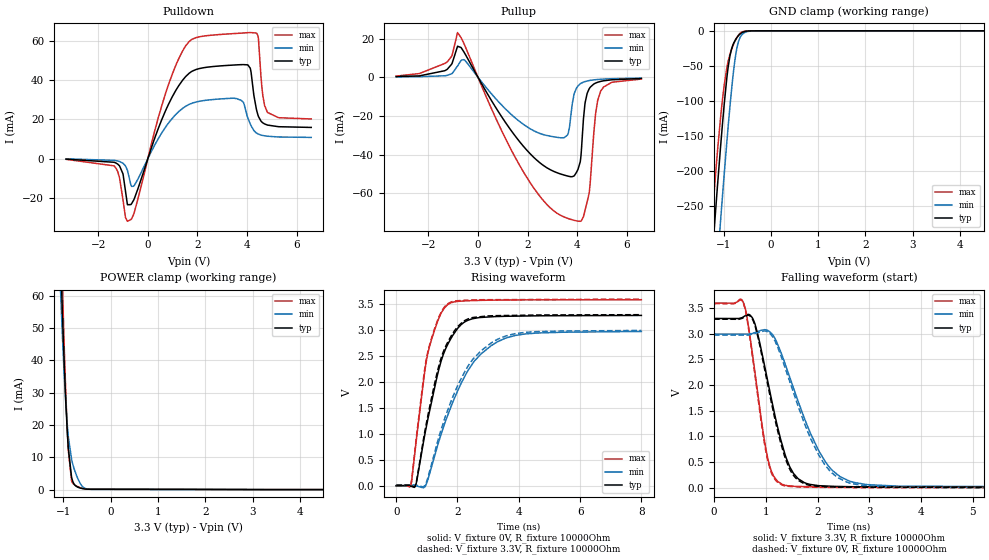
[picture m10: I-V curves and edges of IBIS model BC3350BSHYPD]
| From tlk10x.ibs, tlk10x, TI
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|   Model
[Model]   BC3350BSHYPD
Model_type   I/O
Polarity   Non-Inverting
Enable   Active-Low
Vinl = 0.99
Vinh = 2.31
Vmeas = 1.65
Vref = 1.65
Cref = 1pF
Rref = 10000
|   typ   min   max
C_comp   1.945pF   1.862pF   2.001pF
[Voltage Range]   3.3   3   3.6
[Temperature Range]   25   125   -40
[Pullup Reference]   3.3   3   3.6
[Pulldown Reference]   -0   -0   -0
[Power Clamp Reference]   3.3   3   3.6
[GND Clamp Reference]   -0   -0   -0
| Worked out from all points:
|   slope of the pulldown table from 0 to 0.495 V, typ, clamps not added: 27.8 ohm
|   slope of the pullup table from 0 to 0.495 V, typ, clamps not added: 45 ohm
|   GND clamp passes 1 mA (typ) near -0.55 V on its own axis
|   POWER clamp passes 1 mA (typ) near -0.72 V on its own axis
|   falling waveform, V_fixture 3.3V, R_fixture 10000Ohm: 20-80 % time 445ps typ, 712ps min, 304ps max; typ from 3.29 V to 0.009 V
|   rising waveform, V_fixture 0V, R_fixture 10000Ohm: 20-80 % time 768ps typ, 1.26ns min, 555ps max; typ from 0 V to 3.28 V
|   rising waveform, V_fixture 3.3V, R_fixture 10000Ohm: 20-80 % time 752ps typ, 1.21ns min, 552ps max; typ from 0.009 V to 3.29 V
|   falling waveform, V_fixture 0V, R_fixture 10000Ohm: 20-80 % time 438ps typ, 692ps min, 301ps max; typ from 3.28 V to 0 V
[Pulldown]
|   Voltage   I(typ)   I(min)   I(max)
-3.3V     -306.9uA   -177.2uA   -405.8uA
-1.36V    -1.92mA    -935.1uA   -3.757mA
-904.2mV  -16.59mA   -3.769mA   -30.07mA
-676.5mV  -23.41mA   -13.77mA   -31.09mA
976.8mV   31.4mA     20.44mA    42.88mA
2.224V    46.37mA    29.58mA    62.55mA
3.749V    47.99mA    29.83mA    64.09mA
4.036V    47.8mA     20.63mA    64.34mA
4.392V    24.41mA    12.94mA    64.04mA
4.64V     18.21mA    11.76mA    31.98mA
4.818V    17.14mA    11.41mA    23.72mA
6.59V     15.9mA     10.79mA    20.22mA
[GND Clamp]
|   Voltage   I(typ)   I(min)   I(max)
-3.3V     -2.327A    -2.431A    -2.267A
-1.251V   -331.9mA   -441.7mA   -275.1mA
-1.142V   -233.8mA   -342.1mA   -183mA
-1.063V   -165.7mA   -271.4mA   -124mA
-993.3mV  -110.6mA   -211.3mA   -81.83mA
-933.9mV  -69.64mA   -161.9mA   -54.33mA
-864.6mV  -35.7mA    -108.2mA   -33.42mA
-795.3mV  -19.15mA   -61.62mA   -20.36mA
-735.9mV  -11.53mA   -31.57mA   -11.73mA
-676.5mV  -6.269mA   -13.91mA   -5.467mA
-597.3mV  -2.127mA   -4.66mA    -1.311mA
6.59V     0A         0A         0A
[Pullup]
|   Voltage   I(typ)   I(min)   I(max)
-3.3V     399.3uA    220.7uA    636uA
-1.251V   4.083mA    981.7uA    7.894mA
-825mV    16.09mA    5.87mA     23.18mA
1.531V    -30.93mA   -21.37mA   -42.19mA
3.214V    -49.54mA   -31.12mA   -70.62mA
3.62V     -51.15mA   -29.62mA   -73.07mA
3.868V    -51.13mA   -9.193mA   -74.03mA
4.125V    -43.72mA   -3.369mA   -74.58mA
4.402V    -8.368mA   -1.906mA   -64.53mA
4.749V    -2.95mA    -1.219mA   -18.38mA
4.947V    -2.114mA   -1.008mA   -7.256mA
6.59V     -611.8uA   -409.7uA   -889.8uA
[POWER Clamp]
|   Voltage   I(typ)   I(min)   I(max)
-3.3V     1.546A     1.464A     1.615A
-1.053V   70.26mA    59.72mA    82.03mA
-1.023V   56.57mA    49.11mA    65.71mA
-1.013V   52.27mA    45.78mA    60.51mA
-943.8mV  26.16mA    25.98mA    28.59mA
-894.3mV  12.85mA    16.45mA    12.3mA
-825mV    3.843mA    9.392mA    2.761mA
-775.5mV  1.803mA    6.676mA    1.629mA
-686.4mV  712.3uA    3.218mA    861.3uA
-567.6mV  246uA      612.7uA    302.1uA
-409.2mV  104.2uA    72.07uA    174.6uA
6.59V     0A         0A         0A
[Ramp]
R_load = 10000
|   typ   min   max
dV/dt_r   1.96823/7.68e-10   1.78225/1.25675e-09   2.14992/5.55243e-10
dV/dt_f   1.97183/4.44578e-10   1.78694/7.09211e-10   2.15286/3.04091e-10
[Falling Waveform]
V_fixture = 3.3V
V_fixture_min = 3V
V_fixture_max = 3.6V
R_fixture = 10000Ohm
C_fixture = 0F
|   Time   V(typ)   V(min)   V(max)
0s        3.295V     2.992V     3.595V
573.4ps   3.33V      2.991V     3.59V
792.5ps   3.183V     3.022V     2.23V
1.034ns   2.096V     3.063V     596.5mV
1.15ns    1.535V     2.953V     232.7mV
1.317ns   840.5mV    2.569V     68.16mV
1.538ns   276.7mV    1.935V     31.35mV
2.022ns   43.2mV     728.8mV    17.88mV
2.607ns   23.19mV    135.6mV    13.99mV
8ns       8.614mV    13.35mV    6.723mV
[Rising Waveform]
V_fixture = 0V
V_fixture_min = 0V
V_fixture_max = 0V
R_fixture = 10000Ohm
C_fixture = 0F
|   Time   V(typ)   V(min)   V(max)
0s        318.3uV    1.66mV     54.1uV
461ps     -4.926mV   2.658mV    -15.53mV
633ps     1.635mV    820.2uV    757mV
1.034ns   1.284V     117.8mV    2.552V
1.39ns    2.239V     850.1mV    3.223V
1.674ns   2.714V     1.346V     3.487V
2.125ns   3.107V     1.98V      3.556V
2.518ns   3.22V      2.376V     3.567V
3.567ns   3.264V     2.843V     3.577V
8ns       3.281V     2.972V     3.583V
[Rising Waveform]
V_fixture = 3.3V
V_fixture_min = 3V
V_fixture_max = 3.6V
R_fixture = 10000Ohm
C_fixture = 0F
|   Time   V(typ)   V(min)   V(max)
0s        8.613mV    13.33mV    6.722mV
461ps     3.88mV     14.18mV    -7.081mV
623.2ps   961uV      14mV       747.2mV
884.8ps   878.2mV    -23.42mV   2.042V
1.025ns   1.324V     135.9mV    2.564V
1.372ns   2.265V     894.7mV    3.221V
1.674ns   2.757V     1.445V     3.504V
2.379ns   3.219V     2.337V     3.577V
3.306ns   3.277V     2.821V     3.584V
8ns       3.295V     2.992V     3.595V
[Falling Waveform]
|Gnd
V_fixture = 0V
V_fixture_min = 0V
V_fixture_max = 0V
R_fixture = 10000Ohm
C_fixture = 0F
|   Time   V(typ)   V(min)   V(max)
0s        3.281V     2.972V     3.583V
573.4ps   3.315V     2.972V     3.573V
792.5ps   3.153V     3.005V     2.18V
1.025ns   2.075V     3.038V     593.7mV
1.143ns   1.496V     2.922V     218.1mV
1.317ns   775.2mV    2.501V     54.19mV
1.573ns   196.7mV    1.74V      22.13mV
2ns       30.23mV    684mV      10.67mV
2.558ns   13.74mV    115.3mV    5.968mV
8ns       319.4uV    1.682mV    54.63uV
